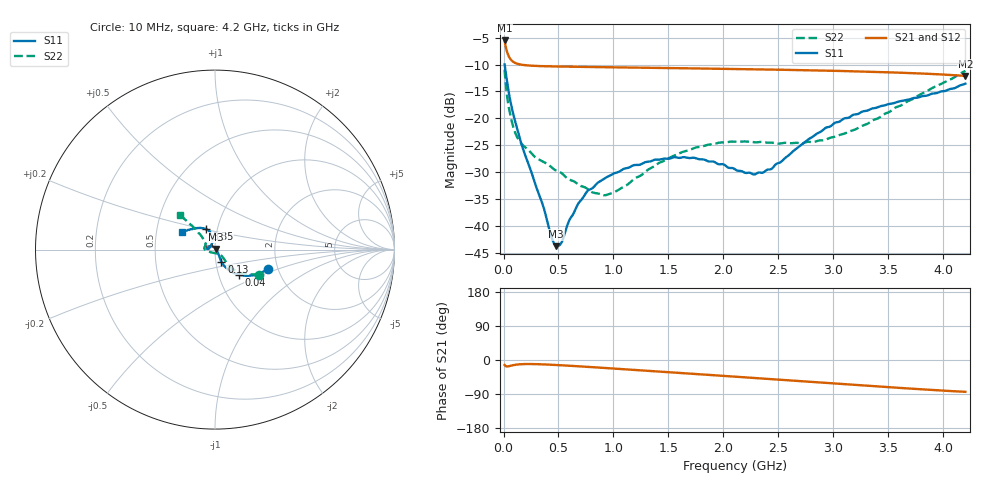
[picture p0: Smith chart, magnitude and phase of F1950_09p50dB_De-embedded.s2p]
! Integrated Device Technology
! Corporate Headquarters
! 6024 Silver Creek Valley Road
! San Jose, CA 95138  USA
! Phone:  1-408-284-8200
! Toll Free:  1-800-223-1366
! Webpage:  http://www.idt.com/
! Timing and RF Division
! 515 Groton Road, Suite 102
! Westford, MA 01886-6024
! Device:  F1950
! Description: 7-bit 0.25 dB Digital Step Attenuator
! Frequency:  150.0 -  4000.00 MHz
! Package:  4x4 mm Thin QFN Plastic Package: 24 pin
! Ports:  2 RF, 12 DC
!  Pin  1  = D0
!  Pin  2  = VDD
!  Pin  3  = Vmode
!  Pin  4  = GND
!  Pin  5  = RF1  =  Port 1
!  Pin  6  = GND
!  Pin  7  = GND
!  Pin  8  = GND
!  Pin  9  = GND
!  Pin 10  = GND
!  Pin 11  = GND
!  Pin 12  = GND
!  Pin 13  = GND
!  Pin 14  = RF2  =  Port 2
!  Pin 15  = GND
!  Pin 16  = LE
!  Pin 17  = CLK
!  Pin 18  = DATE
!  Pin 19  = D6
!  Pin 20  = D5
!  Pin 21  = D4
!  Pin 22  = D3
!  Pin 23  = D2
!  Pin 24  = D1
! State:  38
! Atten State:  9.50 dB
! Voltage:  +5.00 Volts
! Current:  Not Measured mA
! Data:  The device was measured on a the F195X evaluation board which has
!  individual transmission lines to the RF pins.  Data was collected
!  using a calibrated network analyzer.  The evaluation board was
!  de-embedded using a TRL calibration technique.
!  The reference plane is the edge of the package pin.
! Misc:  Board 2019
!  Action Tracker AT0250
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# GHz S dB R 50
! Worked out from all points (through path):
!   420 points, 10 MHz to 4.2 GHz, reference 50 ohm
!   highest |S21| = -5.51 dB at 10 MHz (marker M1); lowest = -12.1 dB at 4.2 GHz (marker M2)
!   group delay of S21, straight-line fit = 52.4 ps
!   lowest |S11| = -43.8 dB at 480 MHz (marker M3), VSWR 1.01, Z = 50.5 + j0.359 ohm
!   |S11| at or under -10 dB: 10.14 MHz to end of sweep
!   |S22| runs from -34.3 to -10.9 dB; largest |S21 - S12| = 0.00038
!   S11 on the Smith chart (normalised r, x): 10 MHz: 1.78, -0.43; 40 MHz: 1.25, -0.37; 130 MHz: 1.06, -0.14; 3.35 GHz: 0.89, +0.20; 4.2 GHz: 0.68, +0.14
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0.01  -9.98 -20.3  -5.51 -13.2  -5.51 -13.2  -10.95 -29.3
0.04  -14.21 -46.1  -8.09 -16.9  -8.09 -16.9  -16.97 -48.1
0.08  -18.49 -58.6  -9.35 -14.2  -9.35 -14.2  -20.98 -48.1
0.13  -22.40 -61.9  -9.87 -11.8  -9.87 -11.8  -23.74 -44.6
0.36  -36.33 -35.3  -10.30 -11.5  -10.30 -11.5  -28.08 -45.2
0.44  -42.35 -2.4  -10.34 -12.6  -10.34 -12.6  -29.19 -46.5
0.48  -43.81 33.4  -10.36 -13.2  -10.36 -13.2  -29.75 -49.5
0.53  -43.05 70.6  -10.38 -14.0  -10.37 -14.0  -30.24 -50.8
0.6  -38.90 100.5  -10.40 -15.1  -10.40 -15.2  -31.43 -56.4
0.71  -35.14 118.1  -10.43 -17.1  -10.43 -17.1  -32.67 -67.4
0.77  -33.41 123.4  -10.45 -18.2  -10.45 -18.2  -33.26 -74.7
0.95  -30.85 138.4  -10.50 -21.5  -10.50 -21.6  -34.19 -107.9
1.41  -27.69 165.7  -10.63 -30.3  -10.62 -30.4  -28.35 -163.4
1.73  -27.35 175.2  -10.71 -36.6  -10.71 -36.6  -25.58 -177.0
2.11  -29.57 166.4  -10.83 -44.1  -10.83 -44.2  -24.37 172.9
2.28  -30.47 145.8  -10.89 -47.5  -10.88 -47.5  -24.46 168.9
2.37  -30.00 132.7  -10.92 -49.3  -10.92 -49.3  -24.45 166.6
2.81  -23.46 101.7  -11.08 -58.0  -11.07 -58.1  -24.44 150.9
3.09  -20.11 104.7  -11.20 -63.7  -11.20 -63.7  -22.92 142.7
3.35  -18.20 113.0  -11.35 -68.8  -11.35 -68.9  -20.48 136.6
3.51  -17.32 118.9  -11.44 -71.9  -11.44 -72.0  -18.81 134.9
4.2  -13.55 151.3  -12.12 -83.9  -12.11 -84.0  -11.17 135.4
